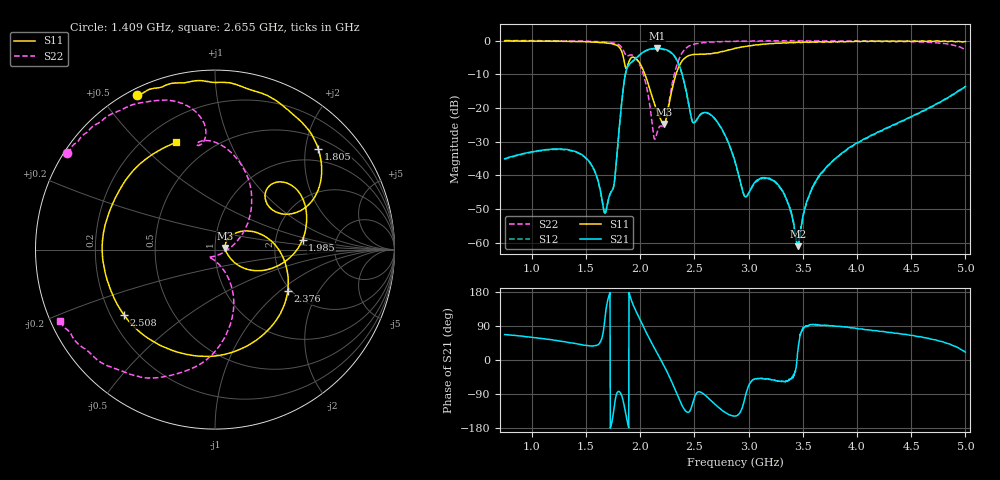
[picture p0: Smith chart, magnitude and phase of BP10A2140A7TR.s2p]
!Agilent Technologies,E8358A,US41080443,A.07.50.56
!Agilent E8358A: A.07.50.56
!Date: Friday, August 07, 2015 14:28:18
!Correction: S11(Full 2 Port(1,2))
!S21(Full 2 Port(1,2))
!S12(Full 2 Port(1,2))
!S22(Full 2 Port(1,2))
!S2P File: Measurements: S11, S21, S12, S22:
# Hz S  dB  R 50
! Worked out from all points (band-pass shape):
!   1601 points, 750 MHz to 5 GHz, reference 50 ohm
!   highest |S21| = -2.33 dB at 2.152 GHz (marker M1); lowest = -61.0 dB at 3.454 GHz (marker M2)
!   |S21| within 3 dB of the highest: 1.959 GHz to 2.332 GHz (372.1 MHz wide, 17.3 % of centre)
!   lowest |S11| = -24.8 dB at 2.219 GHz (marker M3), VSWR 1.12, Z = 56 + j1.02 ohm
!   |S11| at or under -10 dB: 2.044 GHz to 2.331 GHz (287.1 MHz wide, 13.1 % of centre)
!   |S22| runs from -29.3 to 0.0 dB; largest |S21 - S12| = 0.012
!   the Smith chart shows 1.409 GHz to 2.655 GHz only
!   S11 on the Smith chart (normalised r, x): 1.409 GHz: 0.02, +0.61; 1.805 GHz: 0.71, +2.26; 1.985 GHz: 2.86, +0.41; 2.376 GHz: 1.93, -1.13; 2.508 GHz: 0.25, -0.30; 2.655 GHz: 0.32, +0.65
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7.5e8  -0.14 152.0  -35.04 67.1  -35.18 67.2  -0.02 165.6
1.40875e9  -0.30 116.8  -33.00 42.9  -33.11 43.0  -0.14 146.8
1.459219e9  -0.31 112.4  -33.74 40.4  -33.90 40.6  -0.16 144.5
1.679688e9  -0.71 81.1  -50.98 118.9  -51.07 120.5  -0.43 127.8
1.756719e9  -1.13 62.3  -43.10 -133.1  -43.23 -133.2  -0.76 116.8
1.804531e9  -1.89 44.4  -26.90 -83.1  -27.00 -82.7  -1.26 106.4
1.870938e9  -8.31 38.3  -8.98 -147.3  -9.09 -147.0  -4.50 96.9
1.985156e9  -6.18 6.4  -4.52 114.5  -4.67 114.7  -6.46 70.1
2.1525e9  -20.58 -28.3  -2.33 20.5  -2.46 20.6  -27.68 -108.5
2.168438e9  -21.86 -23.7  -2.34 12.2  -2.47 12.3  -26.09 -123.7
2.218906e9  -24.76 9.0  -2.55 -14.6  -2.68 -14.5  -25.51 -111.9
2.375625e9  -6.63 -29.6  -8.74 -113.3  -8.86 -113.2  -4.31 -93.8
2.508438e9  -4.10 -144.1  -24.11 -93.0  -24.22 -92.8  -0.98 -135.2
2.654531e9  -3.93 109.8  -22.10 -107.2  -22.19 -107.5  -0.44 -155.3
2.875e9  -2.32 -8.8  -35.83 -148.2  -36.03 -147.8  -0.26 -170.5
2.970625e9  -1.76 -41.6  -46.34 -95.6  -46.34 -95.3  -0.14 -174.9
3.10875e9  -1.18 -76.0  -40.92 -48.5  -40.93 -48.6  -0.11 179.6
3.310625e9  -0.74 -108.8  -44.58 -56.7  -44.65 -56.6  -0.08 172.5
3.454062e9  -0.53 -124.6  -60.97 22.1  -60.61 18.9  -0.07 167.3
3.584219e9  -0.44 -135.2  -43.89 92.8  -44.02 92.8  -0.08 163.0
4.293438e9  -0.29 -163.6  -25.69 72.9  -25.84 73.1  -0.29 136.8
5e9  -0.31 175.7  -13.61 20.9  -13.73 20.6  -2.68 61.9
